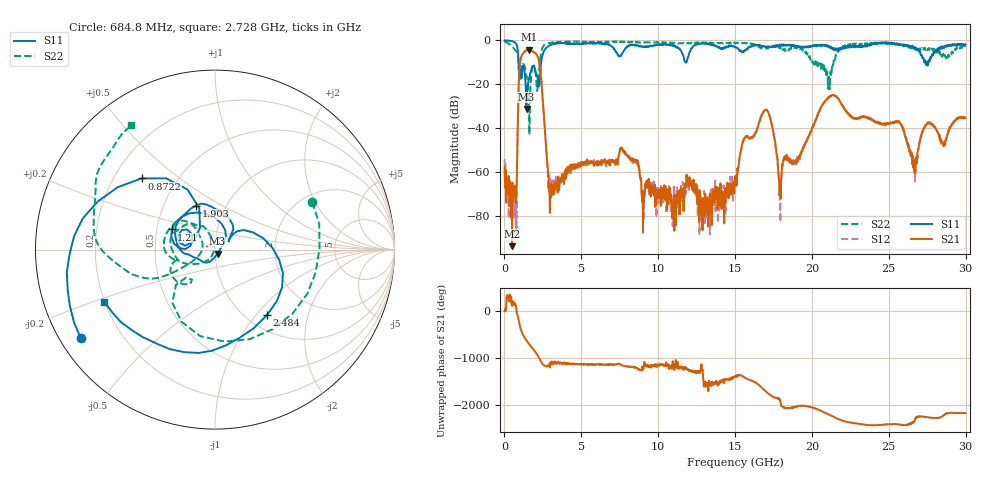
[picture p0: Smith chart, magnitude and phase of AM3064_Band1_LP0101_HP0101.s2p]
# Hz S DB R 50.0
!freq dBS11 angS11 dBS21 angS21 dBS12 angS12 dBS22 angS22
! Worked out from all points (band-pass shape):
!   1600 points, 10 MHz to 29.98 GHz, reference 50 ohm
!   highest |S21| = -4.30 dB at 1.584 GHz (marker M1); lowest = -93.9 dB at 497.3 MHz (marker M2)
!   |S21| within 3 dB of the highest: 1.096 GHz to 2.158 GHz (1.062 GHz wide, 65.2 % of centre)
!   lowest |S11| = -31.3 dB at 1.435 GHz (marker M3), VSWR 1.06, Z = 51.4 - j2.38 ohm
!   |S11| at or under -10 dB: 916.8 MHz to 2.389 GHz (1.472 GHz wide, 89.1 % of centre); 27.39244 GHz to 27.46089 GHz (68.45 MHz wide, 0.25 % of centre); 27.48979 GHz to 27.56406 GHz (74.26 MHz wide, 0.27 % of centre)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
!   |S22| runs from -43.0 to -0.4 dB; largest |S21 - S12| = 0.0085
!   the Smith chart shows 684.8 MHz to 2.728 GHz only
!   S11 on the Smith chart (normalised r, x): 684.8 MHz: 0.06, -0.30; 872.2 MHz: 0.32, +0.37; 1.21 GHz: 0.60, +0.14; 1.903 GHz: 0.72, +0.38; 2.484 GHz: 1.22, -1.14; 2.728 GHz: 0.20, -0.22
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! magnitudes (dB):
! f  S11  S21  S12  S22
! 10 MHz  0.0  -57.9  -54.2  -0.4
! 497.3 MHz  -0.4  -93.9  -73.8  -2.7
! 684.8 MHz  -1.0  -69.3  -67.2  -4.4
! 872.2 MHz  -4.9  -36.1  -36.0  -7.1
! 1.21 GHz  -11.5  -5.9  -5.9  -10.9
! 1.435 GHz  -31.3  -4.5  -4.4  -16.5
! 1.584 GHz  -17.9  -4.3  -4.3  -26.2
! 1.903 GHz  -11.5  -5.4  -5.3  -11.9
! 2.484 GHz  -6.6  -26.4  -26.3  -3.3
! 2.728 GHz  -3.3  -50.9  -49.6  -1.6
! 3.084 GHz  -1.9  -69.3  -68.4  -1.1
! 5.015 GHz  -1.4  -56.4  -56.6  -0.8
! 7.657 GHz  -5.9  -49.4  -50.0  -0.7
! 10 GHz  -2.0  -68.1  -68.2  -0.9
! 15 GHz  -3.0  -64.7  -61.8  -1.4
! 16.92 GHz  -2.9  -31.9  -31.9  -3.6
! 17.91 GHz  -2.0  -68.7  -73.3  -3.3
! 19.99 GHz  -2.9  -40.5  -40.9  -9.4
! 21.34 GHz  -3.7  -25.0  -24.9  -10.8
! 25 GHz  -1.0  -37.8  -37.7  -1.1
! 26.72 GHz  -3.8  -58.7  -59.4  -3.7
! 29.98 GHz  -1.8  -35.3  -35.2  -2.9
